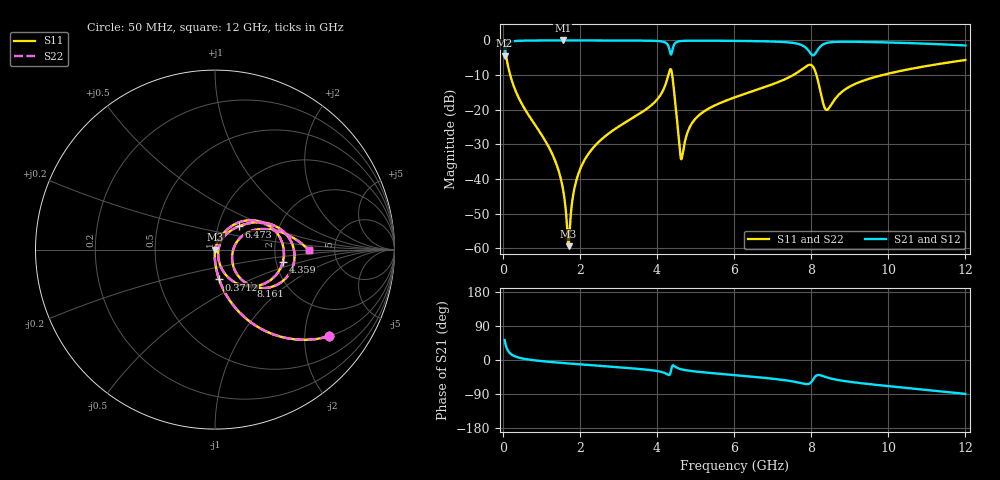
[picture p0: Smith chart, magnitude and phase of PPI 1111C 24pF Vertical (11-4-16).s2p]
# GHz S MA R 50
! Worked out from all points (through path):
!   1601 points, 50 MHz to 12 GHz, reference 50 ohm
!   highest |S21| = -0.01 dB at 1.559 GHz (marker M1); lowest = -4.4 dB at 50 MHz (marker M2)
!   group delay of S21, straight-line fit = 21.2 ps
!   lowest |S11| = -59.4 dB at 1.708 GHz (marker M3), VSWR 1.00, Z = 50.1 - j0.00474 ohm
!   |S11| at or under -10 dB: 195.7 MHz to 4.296 GHz (4.1 GHz wide, 183 % of centre); 4.396 GHz to 7.534 GHz (3.138 GHz wide, 52.6 % of centre); 8.137 GHz to 9.849 GHz (1.711 GHz wide, 19 % of centre)
!   |S22| runs from -59.4 to -2.0 dB; largest |S21 - S12| = 0
!   S11 on the Smith chart (normalised r, x): 50 MHz: 0.99, -2.62; 371.2 MHz: 0.99, -0.34; 4.359 GHz: 2.17, -0.36; 6.473 GHz: 1.25, +0.34; 8.161 GHz: 1.35, -0.59; 12 GHz: 3.18, -0.01
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0.05  0.7971 -37.4  0.6037 52.6  0.6037 52.6  0.7971 -37.4
0.1695  0.3601 -69.7  0.9325 20.2  0.9325 20.2  0.3601 -69.7
0.3711563  0.1675 -82.2  0.9853 7.7  0.9853 7.7  0.1675 -82.2
1.259937  0.02456 -93.2  0.9987 -5.3  0.9987 -5.3  0.02456 -93.2
1.558688  0.007389 -90.0  0.9989 -7.9  0.9989 -7.9  0.007389 -90.0
1.708063  0.001071 -2.5  0.9988 -9.1  0.9988 -9.1  0.001071 -2.5
1.864906  0.007506 71.1  0.9987 -10.3  0.9987 -10.3  0.007506 71.1
2.044156  0.01538 73.9  0.9986 -11.7  0.9986 -11.7  0.01538 73.9
4.038312  0.1479 56.5  0.9791 -29.7  0.9791 -29.7  0.1479 56.5
4.262375  0.2708 37.0  0.8925 -37.5  0.8925 -37.5  0.2708 37.0
4.359469  0.3846 -10.7  0.6291 -30.3  0.6291 -30.3  0.3846 -10.7
4.643281  0.0197 3.6  0.9824 -24.8  0.9824 -24.8  0.0197 3.6
5.024188  0.07667 55.3  0.9913 -30.6  0.9913 -30.6  0.07667 55.3
6.025  0.1512 48.7  0.9843 -39.9  0.9843 -39.9  0.1512 48.7
6.473125  0.1842 44.6  0.9778 -44.0  0.9778 -44.0  0.1842 44.6
7.668125  0.3515 22.8  0.8895 -59.4  0.8895 -59.4  0.3515 22.8
8.019156  0.4355 -17.9  0.6211 -56.4  0.6211 -56.4  0.4355 -17.9
8.161062  0.2831 -45.2  0.7174 -39.8  0.7174 -39.8  0.2831 -45.2
8.415  0.09947 -6.4  0.921 -46.1  0.921 -46.1  0.09947 -6.4
8.975156  0.2116 27.7  0.9581 -57.2  0.9581 -57.2  0.2116 27.7
10.01331  0.3328 19.5  0.9339 -69.1  0.9339 -69.1  0.3328 19.5
12  0.5216 -0.1  0.846 -89.4  0.846 -89.4  0.5216 -0.1
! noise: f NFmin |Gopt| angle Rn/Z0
0.05  0.0003542  0.861  1.124  0.0005461
1.372  0.003558  0.6593  7.394  0.001987
2.701  0.006153  0.6241  14.03  0.003018
4.031  0.01875  0.7993  20.97  0.01872
5.36  0.01409  0.6764  27.42  0.00795
6.682  0.01854  0.6977  33.59  0.01102
8.012  0.1878  0.9599  40.62  0.9299
9.341  0.03181  0.7607  46.08  0.0229
10.67  0.02622  0.6942  50.75  0.01376
12  0.02704  0.6839  55.32  0.01313
